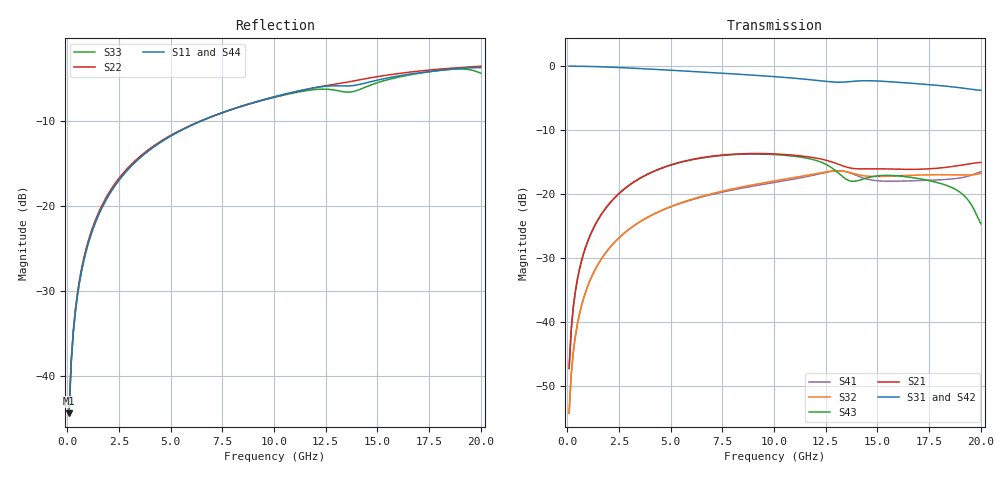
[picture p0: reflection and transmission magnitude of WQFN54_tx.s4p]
! Generated by program util_convert_matmxmd4pspars_to_s4psended on 05-13-2014 07:49:02
!  1 ----xxxxxxxxxxxxxxxxxx---- 3
!  xxxxxxxxxxxxxxxxxx
!  (Input) xxxxxxxxxxxxxxxxxx  (Output)
!  xxxxxxxxxxxxxxxxxx
!  2 ----xxxxxxxxxxxxxxxxxx---- 4
# MHZ S DB R 50.00
! FREQ  S11  S12  S13  S14
!  S21  S22  S23  S24
!  S31  S32  S33  S34
!  S41  S42  S43  S44
!  DB  ANG  DB  ANG  DB  ANG  DB  ANG
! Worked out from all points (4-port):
!   200 points, 100 MHz to 20 GHz, reference 50 ohm
!   strongest paths, dB at 100 MHz, 5.1 GHz, 10.1 GHz, 15.1 GHz, 20 GHz:
!     S31: 0.0, -0.7, -1.7, -2.3, -3.8
!     S42: 0.0, -0.7, -1.7, -2.6, -3.7
!     S21: -47.2, -15.3, -13.7, -16.0, -15.0
!     S43: -47.2, -15.4, -13.8, -17.1, -24.6
!     S32: -54.2, -21.8, -17.9, -17.2, -16.8
!     S41: -54.2, -21.9, -18.1, -17.9, -16.5
!   lowest |S11| = -44.4 dB at 100 MHz (marker M1), VSWR 1.01, Z = 50.1 + j0.595 ohm
!   |S11| at or under -10 dB: start of sweep to 6.45 GHz
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100  -44.37 79.3  -47.20 83.1  -0.01 -0.8  -54.16 -99.2
     -47.20 83.1  -44.02 77.7  -54.19 -98.7  -0.02 -0.9
     -0.01 -0.8  -54.19 -98.7  -44.36 78.5  -47.17 82.9
     -54.16 -99.2  -0.02 -0.9  -47.17 82.9  -44.02 77.1
400  -32.46 84.0  -35.22 84.3  -0.02 -3.3  -42.20 -99.1
     -35.22 84.3  -32.16 83.3  -42.22 -99.2  -0.02 -3.6
     -0.02 -3.3  -42.22 -99.2  -32.47 83.0  -35.19 83.8
     -42.20 -99.1  -0.02 -3.6  -35.19 83.8  -32.17 82.4
1200  -23.02 78.8  -25.82 76.9  -0.07 -9.9  -32.78 -112.4
      -25.82 76.9  -22.74 77.6  -32.80 -112.9  -0.07 -10.6
      -0.07 -9.9  -32.80 -112.9  -23.02 76.1  -25.79 75.4
      -32.78 -112.4  -0.07 -10.6  -25.79 75.4  -22.73 75.2
4700  -12.19 53.5  -15.76 45.6  -0.59 -36.6  -22.37 -169.8
      -15.76 45.6  -12.09 50.5  -22.33 -171.6  -0.64 -39.3
      -0.59 -36.6  -22.33 -171.6  -12.18 43.1  -15.79 39.7
      -22.37 -169.8  -0.64 -39.3  -15.79 39.7  -11.98 40.5
11100  -6.48 16.7  -13.95 7.6  -1.93 -80.1  -17.56 102.5
       -13.95 7.6  -6.50 12.7  -17.33 100.3  -1.90 -85.7
       -1.93 -80.1  -17.33 100.3  -6.60 -5.5  -14.12 -9.9
       -17.56 102.5  -1.90 -85.7  -14.12 -9.9  -6.54 -8.9
18400  -3.91 -20.6  -15.77 17.1  -3.16 -124.2  -17.67 14.5
       -15.77 17.1  -3.78 -30.7  -16.96 14.3  -3.30 -133.5
       -3.16 -124.2  -16.96 14.3  -3.92 -45.5  -18.69 -25.4
       -17.67 14.5  -3.30 -133.5  -18.69 -25.4  -3.95 -51.2
20000  -3.69 -30.5  -15.03 19.0  -3.77 -131.5  -16.47 -2.0
       -15.03 19.0  -3.52 -40.7  -16.75 1.5  -3.69 -143.3
       -3.77 -131.5  -16.75 1.5  -4.35 -56.5  -24.63 -18.3
       -16.47 -2.0  -3.69 -143.3  -24.63 -18.3  -4.00 -61.0
